TYPE ST_Setting :
STRUCT
	(*系统*)
	gcSimulationMode:		BOOL;
	JogVelocity:			REAL:=20;
	AutoVelocity:			REAL:=500;(*皮带的速度*)
	ClampVelocity:			REAL:=2000;(*机械手的速度*)

	tCutTime:				REAL:=0.5;(*剪断时间*)

	ZPickUpHeight:			REAL:=200;(*抓起来的高度*)
	XPlacePos:				REAL:=450;(*抓过去的X距离*)
	YPlacePos:				REAL:=330;(*抓过去的Y距离*)
	ZPlacePos:				REAL:=-650;(*放到地板的高度*)
	Box_Longth:				REAL:=215;(*箱子长*)
	Box_Width:				REAL:=190;(*箱子宽*)
	Box_Height:				REAL:=198;(*箱子高*)

END_STRUCT
END_TYPE
